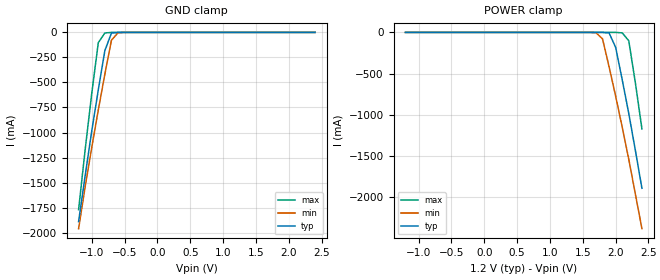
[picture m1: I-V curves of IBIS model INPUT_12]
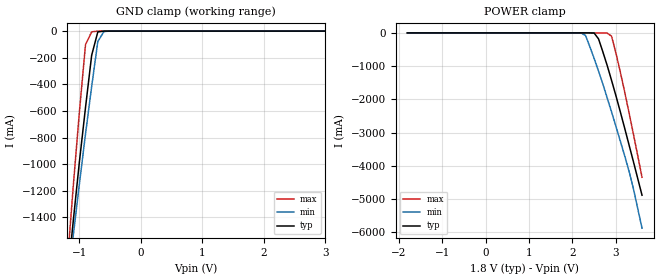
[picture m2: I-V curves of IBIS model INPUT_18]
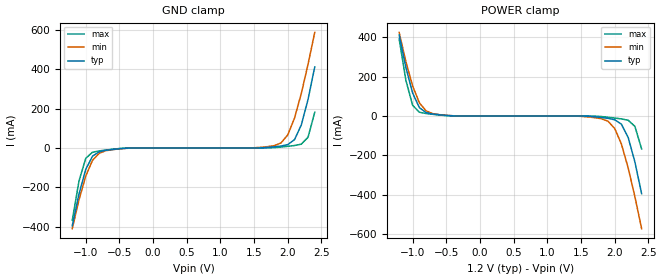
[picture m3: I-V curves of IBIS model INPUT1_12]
|   DIODES INCORPORATED
|   IBIS Model of PI4ULS3V4857
|   Product Family: 4ULS3V
|   WLCSP-20 Package (TBD)
[IBIS Ver] 3.2
[Comment char] |_char
[File Name] pi4uls3v4857_ge_revb.ibs
[File Rev] 1.1
[Source] File originated at Diodes Incorporated.
[Date] 02/28/2020
[Disclaimer] (C) Copyright DIODES INCORPORATED
   All rights reserved
  Diodes Incorporated hereby grants the user of
  this IBIS model a non-exclusive, nontransferable license to
  use this IBIS model under the following terms.
  This IBIS model is provided on an "AS IS" basis and Diodes
  makes absolutely no warranty with respect to the information
  contained herein. DIODES DISCLAIMS AND CUSTOMER WAIVES ALL
  WARRANTIES, EXPRESSED OR IMPLIED, INCLUDING WARRANTIES OF
  MERCHANTABILITY OR FITNESS FOR A PARTICULAR PURPOSE. The
  entire risk as to quality and performance is with the customer.
  Accordingly, in no event shall the company be liable for any
  damages, whether in contract or tort, including any lost
  profits or other incidental, consequential, exemplary, or
  punitive damages arising out of the use or application of the
  IBIS model provided in this package. Further, Diodes reserves
  the right to make changes without notice to any product herein
  to improve reliability, function, or design. Diodes does not
  convey any license under patent rights or any other intellectual
  property rights, including those of third parties.
  The user is granted this license only to use the IBIS model
  and is not granted rights to sell, load, rent, lease or license
  the IBIS model in whole or in part, or in modified form to anyone
  other than user. User may modify the IBIS model to suit its specific
  application but rights to derivative works and such modifications
  shall belong to Diodes.
  Diodes is not obligated to provide maintenance or support
  for the licensed IBIS model.
  Contact Diodes at ATTN: APPLICATION ENGINEERING / IBIS MODELS
  1545 Barber Ln. Milpitas, CA 95035
[Component] pi4uls3v4857
[Manufacturer] Diodes Incorporated.
[Package]
| variable   typ   min  max
R_pkg   0.00000ohm   NA   NA
L_pkg   0.00000nH   NA   NA
C_pkg   0.05000pF   NA   NA
[Pin]   signal_name   model_name   R_pin   L_pin   C_pin
A1   DAT2A   INOUTA   NA   NA   NA
A2   VCCA   POWER   NA   NA   NA
A3   VSD   POWER   NA   NA   NA
A4   DAT2B   INOUTB   NA   NA   NA
B1   DAT3A   INOUTA   NA   NA   NA
B2   CD   INPUT   NA   NA   NA
B3   VCCB   POWER   NA   NA   NA
B4   DAT3B   INOUTB   NA   NA   NA
C1   CMDA   INOUTA   NA   NA   NA
C2   GND   GND   NA   NA   NA
C3   GND   GND   NA   NA   NA
C4   CMDB   INOUTB   NA   NA   NA
D1   DAT0A   INOUTA   NA   NA   NA
D2   CLKA   INPUT1   NA   NA   NA
D3   CLKB   OUTPUT   NA   NA   NA
D4   DAT0B   INOUTB   NA   NA   NA
E1   DAT1A   INOUTA   NA   NA   NA
E2   CLK_FB   OUTPUT1   NA   NA   NA
E3   SEL   INPUT2   NA   NA   NA
E4   DAT1B   INOUTB   NA   NA   NA
[Model Selector] INPUT
INPUT_12   1.2 volt VCCA
INPUT_18   1.8 volt VCCA
[Model Selector] INPUT1
INPUT1_12   1.2 volt VCCA
INPUT1_18   1.8 volt VCCA
[Model Selector] INPUT2
INPUT2_12   1.2 volt VCCA
INPUT2_18   1.8 volt VCCA
[Model Selector] OUTPUT
OUTPUT_LDO   SEL=HIGH
OUTPUT_VSD   SEL=LOW
[Model Selector] OUTPUT1
OUTPUT1_12   1.2 volt VCCA
OUTPUT1_18   1.8 volt VCCA
[Model Selector] INOUTA
INOUTA_12   1.2 volt VCCA
INOUTA_18   1.8 volt VCCA
[Model Selector] INOUTB
INOUTB_LDO   SEL=HIGH
INOUTB_VSD   SEL=LOW
| Models and submodels in the file (22): INPUT_12 (Input), INPUT_18 (Input), INPUT1_12 (Input), INPUT1_18 (Input), INPUT2_12 (Input), INPUT2_18 (Input), OUTPUT_LDO (Output), OUTPUT_VSD (Output), OUTPUT1_12 (Output), OUTPUT1_18 (Output), INOUTA_12 (I/O), IOA_12_1 (Open_source), IOA_12_2 (Open_sink), INOUTA_18 (I/O), IOA_18_1 (Open_source), IOA_18_2 (Open_sink), INOUTB_LDO (I/O), IOB_LDO_1 (Open_source), IOB_LDO_2 (Open_sink), INOUTB_VSD (I/O), IOB_VSD_1 (Open_source), IOB_VSD_2 (Open_sink)
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|   Model INPUT
[Model] INPUT_12
Model_type Input
Vinl = 0.24V
Vinh = 0.96V
| variable   typ   min   max
C_comp   0.131pF   0.130pF   0.132pF
[Voltage Range]   1.2V   1.1V   1.3V
[GND Clamp Reference]   0.000V   0.000V   0.000V
[POWER Clamp Reference]   1.2V   1.1V   1.3V
[temperature range]   40   85   -40
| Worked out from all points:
|   GND clamp passes 1 mA (typ) near -0.61 V on its own axis
[GND Clamp]
| Voltage   I(typ)   I(min)   I(max)
-1.2V     -1.89A     -1.96A     -1.77A
-1.1V     -1.43A     -1.54A     -1.17A
-1V       -985mA     -1.15A     -611mA
-900mV    -574mA     -774mA     -102mA
-800mV    -182mA     -417mA     -5.78mA
-700mV    -6.54mA    -78.3mA    -102uA
-600mV    -196uA     -3.38mA    -11.5uA
2.4V      21.2pA     230pA      14.7pA
[POWER Clamp]   |Note: Vtable = Vcc - Voutput
| Voltage   I(typ)   I(min)   I(max)
-1.2V     12uA       12.1uA     11.7uA
1.7V      -29.1uA    -3.4mA     -16.7uA
1.8V      -214uA     -78.4mA    -21uA
1.9V      -6.56mA    -417mA     -30uA
2V        -182mA     -774mA     -121uA
2.1V      -574mA     -1.15A     -5.8mA
2.2V      -985mA     -1.54A     -102mA
2.3V      -1.43A     -1.96A     -611mA
2.4V      -1.89A     -2.38A     -1.17A
[Model] INPUT_18
Model_type Input
Vinl = 0.36V
Vinh = 1.44V
| variable   typ   min   max
C_comp   0.131pF   0.130pF   0.132pF
[Voltage Range]   1.8V   1.6V   2.0V
[GND Clamp Reference]   0.000V   0.000V   0.000V
[POWER Clamp Reference]   1.8V   1.6V   2.0V
[temperature range]   40   85   -40
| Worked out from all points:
|   GND clamp passes 1 mA (typ) near -0.61 V on its own axis
[GND Clamp]
| Voltage   I(typ)   I(min)   I(max)
-1.8V     -4.88A     -4.67A     -5.7A
-1.2V     -1.89A     -1.96A     -1.77A
-1.1V     -1.43A     -1.54A     -1.17A
-1V       -985mA     -1.15A     -611mA
-900mV    -574mA     -774mA     -102mA
-800mV    -182mA     -417mA     -5.78mA
-700mV    -6.54mA    -78.3mA    -102uA
-600mV    -196uA     -3.38mA    -11.5uA
3.6V      29.3pA     259pA      21.7pA
[POWER Clamp]   |Note: Vtable = Vcc - Voutput
| Voltage   I(typ)   I(min)   I(max)
-1.8V     18uA       18.1uA     17.6uA
2.1V      -21.1uA    -172uA     -20.5uA
2.2V      -23.6uA    -3.41mA    -21.5uA
2.3V      -35.1uA    -78.4mA    -22.5uA
2.5V      -6.57mA    -774mA     -27.8uA
2.6V      -182mA     -1.15A     -36.9uA
2.8V      -985mA     -1.96A     -5.8mA
2.9V      -1.43A     -2.38A     -102mA
3.1V      -2.37A     -3.25A     -1.17A
3.3V      -3.36A     -4.15A     -2.39A
3.4V      -3.86A     -4.67A     -3.03A
3.6V      -4.88A     -5.87A     -4.34A
[Model] INPUT1_12
Model_type Input
Vinl = 0.24V
Vinh = 0.96V
| variable   typ   min   max
C_comp   6.125pF   6.085pF   6.174pF
[Voltage Range]   1.2V   1.1V   1.3V
[GND Clamp Reference]   0.000V   0.000V   0.000V
[POWER Clamp Reference]   1.2V   1.1V   1.3V
[temperature range]   40   85   -40
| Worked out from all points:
|   GND clamp passes 1 mA (typ) near -0.38 V on its own axis
|   POWER clamp passes 1 mA (typ) near -0.41 V on its own axis
[GND Clamp]
| Voltage   I(typ)   I(min)   I(max)
-1.2V     -396mA     -411mA     -368mA
-1.1V     -234mA     -264mA     -168mA
-1V       -109mA     -143mA     -52.6mA
-900mV    -41.8mA    -63.2mA    -21.6mA
-800mV    -19.1mA    -26.5mA    -14.8mA
-400mV    -1.24mA    -1.75mA    -426uA
1.9V      9.98mA     26mA       4.94mA
2V        17.2mA     67.2mA     8.62mA
2.1V      42.8mA     153mA      12.7mA
2.2V      117mA      277mA      19.3mA
2.3V      247mA      426mA      54.6mA
2.4V      413mA      589mA      182mA
[POWER Clamp]   |Note: Vtable = Vcc - Voutput
| Voltage   I(typ)   I(min)   I(max)
-1.2V     413mA      426mA      393mA
-1.1V     247mA      277mA      182mA
-1V       117mA      153mA      54.6mA
-900mV    42.8mA     67.2mA     19.3mA
-800mV    17.2mA     26mA       12.7mA
-400mV    838uA      1.25mA     260uA
1.9V      -11.8mA    -26.5mA    -6.28mA
2V        -19.1mA    -63.2mA    -10.4mA
2.1V      -41.8mA    -143mA     -14.8mA
2.2V      -109mA     -264mA     -21.6mA
2.3V      -234mA     -411mA     -52.6mA
2.4V      -396mA     -574mA     -168mA
